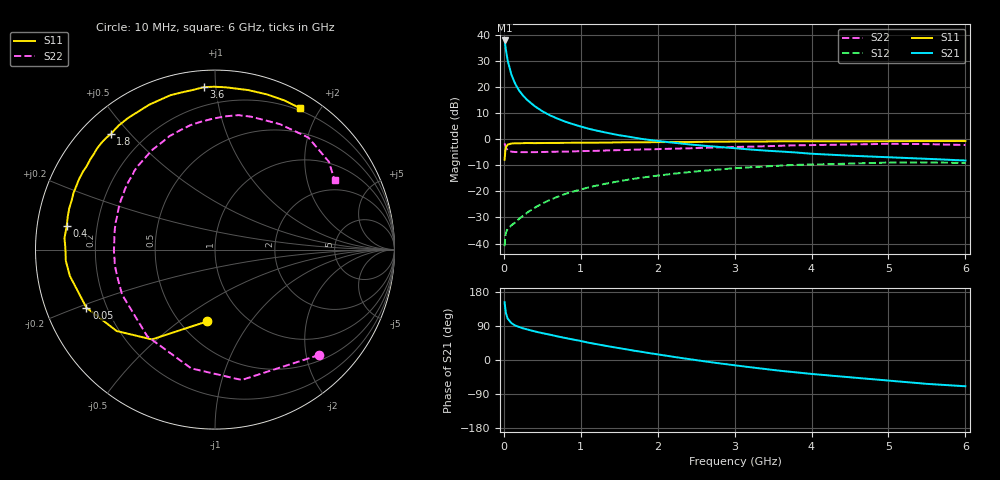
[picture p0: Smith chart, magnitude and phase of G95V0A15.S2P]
! SIEMENS Small Signal Semiconductors
! BFG235
! Si NPN RF Bipolar Junction Transistor in SOT223
! VCE = 5 V  IC = 150 mA
! Common Emitter S-Parameters:  July  1994
# GHz  S  MA  R  50
!  f  S11  S21  S12  S22
! GHz  MAG  ANG  MAG  ANG  MAG  ANG  MAG  ANG
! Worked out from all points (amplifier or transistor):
!   40 points, 10 MHz to 6 GHz, reference 50 ohm
!   highest |S21| = 37.8 dB at 10 MHz (marker M1)
!   |S21| within 3 dB of that: start of sweep to 24.41 MHz
!   unconditionally stable (mu >= 1): 454.9 MHz to 1.458 GHz
!   at 200 MHz: K = 0.81, MSG = 24.5 dB, |S12| = -30.5 dB
!   at 1.5 GHz: K = 0.99, MSG = 8.8 dB, |S12| = -16.1 dB
!   at 6 GHz: K = 0.89, MSG = 0.5 dB, |S12| = -9.2 dB
!   S11 on the Smith chart (normalised r, x): 10 MHz: 0.67, -0.64; 50 MHz: 0.13, -0.21; 400 MHz: 0.09, +0.08; 1.8 GHz: 0.09, +0.44; 3.6 GHz: 0.09, +0.93; 6 GHz: 0.17, +1.75
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0.01  0.4028 -96.4  77.44 152.5  0.0089 62.1  0.8255 -45.3
0.02  0.6118 -125.1  61.06 133.5  0.0141 48.9  0.7415 -78.4
0.03  0.7114 -140.4  47.81 121.7  0.0166 41.8  0.675 -101.3
0.05  0.786 -155.7  31.85 109.1  0.0192 35.1  0.6129 -128.0
0.1  0.8219 -169.7  16.83 97.0  0.0224 37.4  0.5752 -154.1
0.15  0.8335 -175.7  11.29 90.9  0.0255 43.8  0.5651 -165.1
0.2  0.8329 -179.1  8.448 87.1  0.0299 47.9  0.5648 -171.1
0.25  0.8357 178.0  6.807 83.6  0.034 51.6  0.5619 -175.4
0.3  0.8411 175.7  5.686 80.9  0.0387 54.3  0.5632 -178.9
0.4  0.8366 171.1  4.279 75.5  0.0484 57.0  0.5626 176.0
0.5  0.8403 167.7  3.415 70.9  0.0585 58.3  0.5664 171.8
0.7  0.8444 160.9  2.457 62.2  0.0788 57.8  0.5738 164.4
0.9  0.8498 155.5  1.927 54.0  0.0987 54.9  0.5815 158.2
1.1  0.8543 149.2  1.583 45.7  0.1186 51.6  0.5927 152.1
1.4  0.8598 141.8  1.267 34.7  0.1465 45.6  0.6095 143.7
1.8  0.8671 132.0  1.005 21.3  0.1829 37.1  0.6338 132.8
2.2  0.8789 123.4  0.853 8.5  0.2164 28.2  0.6563 122.1
3.2  0.8953 101.9  0.633 -19.0  0.2885 5.0  0.7167 96.3
3.6  0.9072 93.9  0.578 -28.6  0.3104 -4.9  0.7451 85.3
4.5  0.9078 78.2  0.481 -45.6  0.3396 -24.7  0.7872 62.6
5.5  0.9167 64.9  0.419 -63.0  0.3585 -46.5  0.8014 37.6
6  0.9194 59.1  0.389 -69.3  0.3485 -54.8  0.7707 30.2
